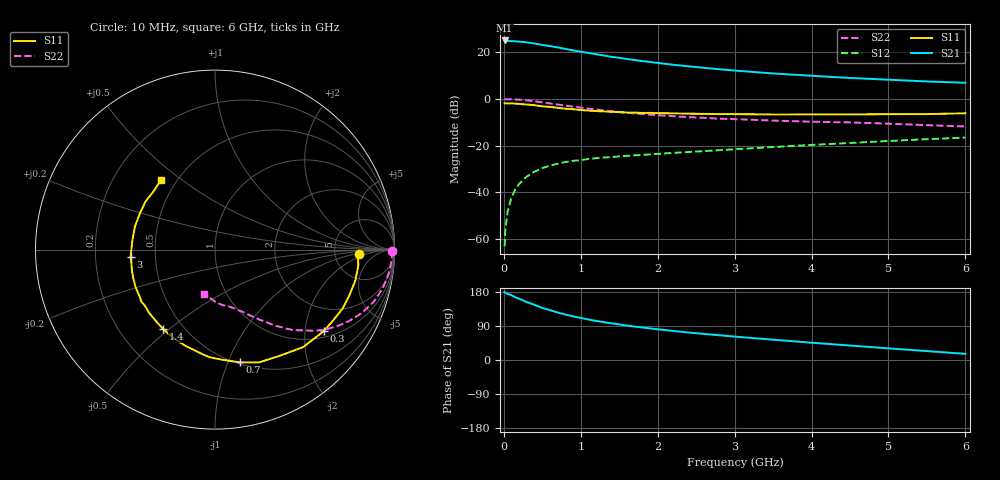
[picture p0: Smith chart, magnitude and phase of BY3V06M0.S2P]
! SIEMENS Small Signal Semiconductors
! BFY420
! Si NPN RF SIEGET Grounded Emitter Transistor in MICRO-X
! VCE = 3 V  IC = 6 mA
! Common Emitter S-Parameters:  October  1996
# GHz  S  MA  R  50
!  f  S11  S21  S12  S22
! GHz  MAG  ANG  MAG  ANG  MAG  ANG  MAG  ANG
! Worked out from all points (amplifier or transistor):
!   36 points, 10 MHz to 6 GHz, reference 50 ohm
!   highest |S21| = 25.0 dB at 10 MHz (marker M1)
!   |S21| within 3 dB of that: start of sweep to 704.1 MHz
!   unconditionally stable (mu >= 1): 3.017 GHz to end of sweep
!   at 250 MHz: K = 0.15, MSG = 29.5 dB, |S12| = -34.7 dB
!   at 1.4 GHz: K = 0.58, MSG = 21.5 dB, |S12| = -24.9 dB
!   at 6 GHz: K = 1.12, MAG = 9.6 dB, |S12| = -16.6 dB
!   S11 on the Smith chart (normalised r, x): 10 MHz: 9.09, -1.16; 300 MHz: 1.18, -2.51; 700 MHz: 0.52, -1.11; 1.4 GHz: 0.39, -0.48; 3 GHz: 0.36, -0.04; 6 GHz: 0.41, +0.42
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0.01  0.8047 -1.6  17.85 179.6  0.0007 77.6  0.9868 -0.5
0.02  0.797 -2.8  17.78 177.4  0.0016 93.2  0.9848 -1.2
0.05  0.8036 -6.3  17.39 174.5  0.0039 85.7  0.9868 -3.1
0.1  0.8006 -12.6  17.3 170.9  0.0078 81.3  0.9809 -6.4
0.15  0.7905 -18.8  17.07 165.3  0.0116 77.3  0.9717 -9.5
0.2  0.7828 -24.9  16.83 161.7  0.0151 76.4  0.9605 -12.5
0.3  0.7574 -36.9  16.22 152.7  0.0218 71.6  0.9297 -18.4
0.4  0.7321 -47.9  15.34 145.5  0.0277 65.7  0.8879 -23.7
0.5  0.6931 -58.6  14.32 137.5  0.0328 62.6  0.8449 -28.2
0.6  0.6747 -68.7  13.53 131.4  0.0373 58.2  0.8009 -32.3
0.7  0.6439 -77.4  12.68 125.4  0.041 55.2  0.7591 -35.9
0.9  0.6006 -93.0  10.94 115.1  0.0472 49.7  0.6811 -41.4
1.1  0.5615 -106.9  9.663 106.9  0.0516 46.6  0.6192 -46.2
1.4  0.5282 -123.2  7.958 96.7  0.0567 43.8  0.5457 -51.3
1.6  0.5112 -133.3  7.143 90.7  0.0603 42.1  0.5039 -54.1
1.8  0.5005 -141.0  6.458 85.8  0.0629 41.5  0.4741 -56.4
2.2  0.4895 -154.6  5.385 76.7  0.0696 40.3  0.427 -60.8
3  0.4714 -175.3  4.05 61.8  0.0834 38.9  0.368 -68.0
3.5  0.4633 173.5  3.506 53.6  0.093 37.7  0.3431 -72.3
4.5  0.4642 154.5  2.808 38.2  0.1137 33.4  0.3131 -81.8
5.5  0.4725 135.8  2.364 23.5  0.1372 27.4  0.2735 -95.0
6  0.4915 127.7  2.212 16.2  0.1485 24.0  0.2567 -103.2
